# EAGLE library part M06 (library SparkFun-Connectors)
Header 6 Standard 6-pin 0.1" header. Use with straight break away headers (SKU : PRT-00116), right angle break away headers (PRT-00553), swiss pins (PRT-00743), machine pins (PRT-00117), and female headers (PRT-00115). Molex polarized connector foot print use with SKU : PRT-08094 with associated crimp pins and housings. NOTES ON THE VARIANTS LOCK and LOCK_LONGPADS... This footprint was designed to help hold the alignment of a through-hole component (i.e. 6-pin header) while soldering it into place. You may notice that each hole has been shifted either up or down by 0.005 of an inch from it's more standard position (which is a perfectly straight line). This slight alteration caused the pins (the squares in the middle) to touch the edges of the holes. Because they are alternating, it causes a "brace" to hold the component in place. 0.005 has proven to be the perfect amount of "off-center" position when using our standard breakaway headers. Although looks a little odd when you look at the bare footprint, once you have a header in there, the alteration is very hard to notice. Also, if you push a header all the way into place, it is covered up entirely on the bottom side. This idea of altering the position of holes to aid alignment will be further integrated into the Sparkfun Library for other footprints. It can help hold any component with 3 or more connection pins.
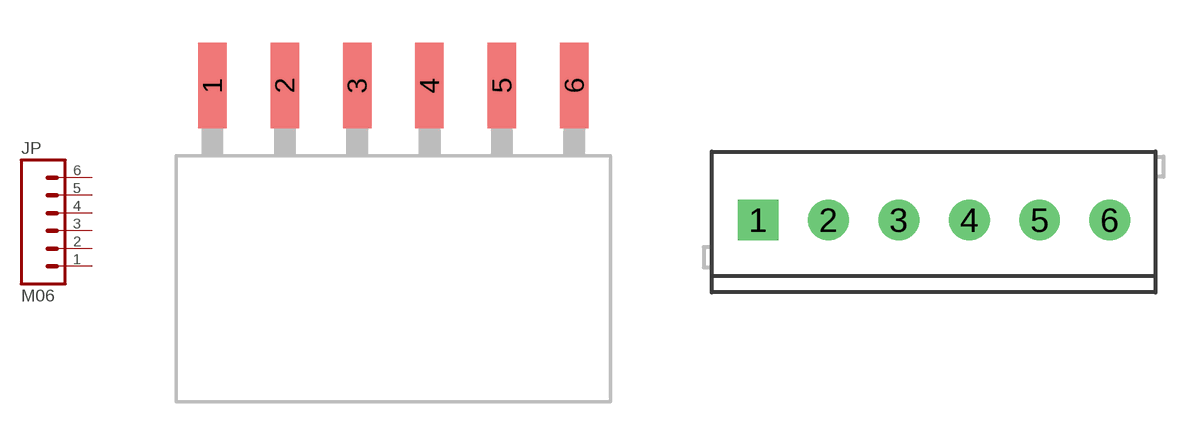
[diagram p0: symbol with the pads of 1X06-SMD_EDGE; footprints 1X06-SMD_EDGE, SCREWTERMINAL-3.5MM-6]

Designator prefix JP

## M061X06-SMD_EDGE_FEMALE  [1X06-SMD_EDGE]
1  1  pas
2  2  pas
3  3  pas
4  4  pas
5  5  pas
6  6  pas

## M063.5MM-6  [SCREWTERMINAL-3.5MM-6]
Pads as for 1X06-SMD_EDGE

## M06EM406  [EM406]
Pads as for 1X06-SMD_EDGE

## M06FEMALE_LOCK  [1X06_FEMALE_LOCK.010]
Pads as for 1X06-SMD_EDGE

## M06LOCK  [1X06_LOCK]
Pads as for 1X06-SMD_EDGE

## M06LOCK_LONGPADS  [1X06_LOCK_LONGPADS]
Pads as for 1X06-SMD_EDGE

## M06LONGPADS  [1X06_LONGPADS]
Pads as for 1X06-SMD_EDGE

## M06POGOPIN_HOLES_ONLY  [1X06_HOLES_ONLY]
Pads as for 1X06-SMD_EDGE

## M06POLAR  [MOLEX-1X6]
Pads as for 1X06-SMD_EDGE

## M06POLAR_LOCK  [MOLEX-1X6_LOCK]
Pads as for 1X06-SMD_EDGE

## M06RA  [MOLEX-1X6-RA]
Pads as for 1X06-SMD_EDGE

## M06RA_LOCK  [MOLEX-1X6-RA_LOCK]
Pads as for 1X06-SMD_EDGE

## M06SIP  [1X06]
Pads as for 1X06-SMD_EDGE

## M06SIP_LOCK  [1X06-SIP_LOCK]
Pads as for 1X06-SMD_EDGE

## M06SMD  [1X06-SMD]
Pads as for 1X06-SMD_EDGE

## M06SMD-FEMALE-V2  [1X06-SMD-FEMALE-V2]
Pads as for 1X06-SMD_EDGE

## M06SMD-STRAIGHT  [1X06_SMD_STRAIGHT]
Pads as for 1X06-SMD_EDGE

## M06SMD-STRAIGHT-ALT  [1X06_SMD_STRAIGHT_ALT]
Pads as for 1X06-SMD_EDGE

## M06SMD-STRAIGHT-COMBO  [1X06_SMD_STRAIGHT_COMBO]
Pads as for 1X06-SMD_EDGE

## M06SMDF  [1X06-SMD-FEMALE]
Pads as for 1X06-SMD_EDGE

## Footprint 1X06-SMD_EDGE (pad centres in mm)
smd 1 x 3: 1 0,-0.08; 2 2.54,-0.08; 3 5.08,-0.08; 4 7.62,-0.08; 5 10.16,-0.08; 6 12.7,-0.08

## Footprint SCREWTERMINAL-3.5MM-6 (pad centres in mm)
drill 1.2 pad 2.032 square: 1 0,0
drill 1.2 pad 2.032: 2 3.5,0; 3 7,0; 4 10.5,0; 5 14,0; 6 17.5,0

## Footprint EM406 (pad centres in mm)
smd 0.6 x 1.55: 1 0,0; 2 1,0; 3 2,0; 4 3,0; 5 4,0; 6 5,0
smd 1.2 x 1.8: P$1 -1.3,-2.225; P$2 6.3,-2.225

## Footprint 1X06_FEMALE_LOCK.010 (pad centres in mm)
drill 1.016 pad 1.88: 1 0,0.254; 2 2.54,-0.254; 3 5.08,0.254; 4 7.62,-0.254; 5 10.16,0.254; 6 12.7,-0.254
